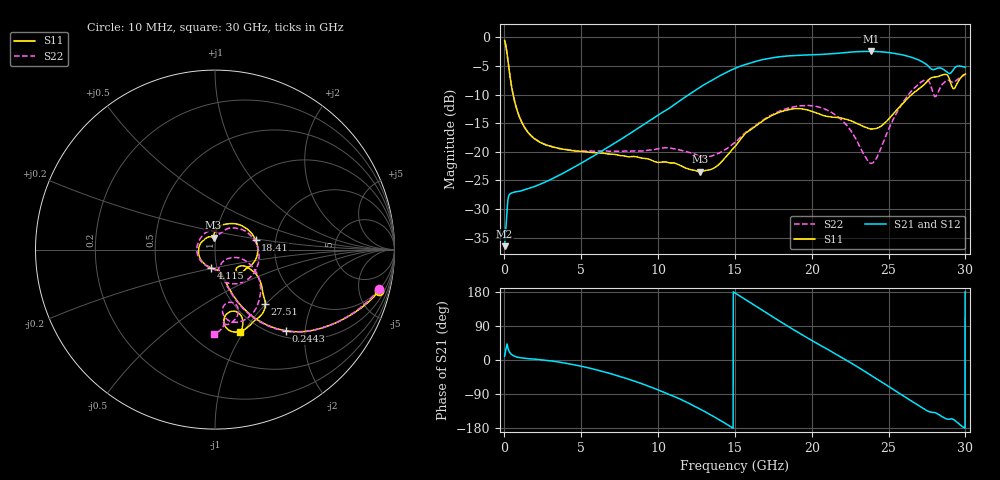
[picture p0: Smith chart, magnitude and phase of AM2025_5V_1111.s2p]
!Keysight Technologies,N5245B,MY58422270,A.16.20.02
!Date: Tuesday, July 14, 2026 01:15:57
!Correction: S11(C  2-Port  )
!S21(C  2-Port  )
!S12(C  2-Port  )
!S22(C  2-Port  )
!S2P File: Measurements: S11, S21, S12, S22:
# Hz S  dB  R 50
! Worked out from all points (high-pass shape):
!   3201 points, 10 MHz to 30 GHz, reference 50 ohm
!   highest |S21| = -2.43 dB at 23.83 GHz (marker M1); lowest = -36.5 dB at 10 MHz (marker M2)
!   |S21| within 3 dB of the highest: 14.98 GHz to 27.75 GHz (12.76 GHz wide, 59.7 % of centre); 29.26 GHz to end of sweep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
!   lowest |S11| = -23.5 dB at 12.73 GHz (marker M3), VSWR 1.14, Z = 48.8 + j6.5 ohm
!   |S11| at or under -10 dB: 563.4 MHz to 26.49 GHz (25.93 GHz wide, 192 % of centre)
!   |S22| runs from -22.0 to -0.5 dB; largest |S21 - S12| = 0.0074
!   S11 on the Smith chart (normalised r, x): 10 MHz: 1.84, -7.53; 244.3 MHz: 1.12, -1.59; 4.115 GHz: 0.94, -0.19; 18.41 GHz: 1.57, +0.18; 27.51 GHz: 1.37, -0.99; 30 GHz: 0.81, -0.97
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1e7  -0.52 -14.3  -36.50 9.9  -39.54 36.9  -0.54 -13.6
2.442969e8  -4.43 -48.9  -28.08 28.9  -28.12 28.8  -4.45 -49.2
3.84875e8  -7.25 -60.2  -27.32 17.6  -27.28 16.9  -7.26 -60.6
5.723125e8  -10.11 -66.6  -27.09 11.4  -27.09 10.9  -10.11 -67.2
1.406409e9  -16.15 -73.0  -26.54 4.2  -26.56 4.3  -16.12 -74.5
4.114881e9  -19.66 -102.5  -23.31 -9.6  -23.28 -9.6  -19.61 -108.9
5.014581e9  -19.92 -118.0  -21.96 -16.7  -21.94 -16.6  -19.82 -126.1
1.000979e10  -21.86 140.0  -13.58 -79.0  -13.57 -79.0  -19.47 126.2
1.272763e10  -23.50 96.9  -8.70 -129.3  -8.70 -129.3  -20.80 75.4
1.5005e10  -19.06 86.2  -5.40 177.0  -5.40 176.9  -18.33 63.5
1.65701e10  -15.05 55.0  -4.02 136.9  -4.02 136.9  -14.94 40.2
1.840699e10  -12.68 13.5  -3.24 90.1  -3.24 90.0  -12.42 2.0
2.000958e10  -12.92 -19.1  -3.03 51.4  -3.03 51.4  -11.96 -32.5
2.209951e10  -14.22 -40.7  -2.66 3.3  -2.66 3.2  -14.86 -73.9
2.383331e10  -16.02 -41.5  -2.43 -39.7  -2.44 -39.7  -22.00 -53.9
2.500479e10  -14.29 -28.9  -2.63 -69.9  -2.62 -70.0  -16.03 -19.0
2.61669e10  -10.87 -32.6  -3.21 -100.1  -3.22 -100.1  -10.45 -34.5
2.750708e10  -7.72 -47.0  -4.80 -133.9  -4.81 -134.0  -7.45 -71.8
2.806002e10  -6.92 -59.8  -5.51 -139.5  -5.52 -139.5  -10.33 -74.8
2.902532e10  -7.81 -82.9  -6.26 -155.5  -6.25 -155.6  -7.66 -83.4
2.932522e10  -8.78 -71.4  -5.25 -159.8  -5.25 -159.9  -7.70 -83.2
3e10  -6.39 -72.9  -5.22 179.7  -5.20 179.6  -6.57 -90.4
